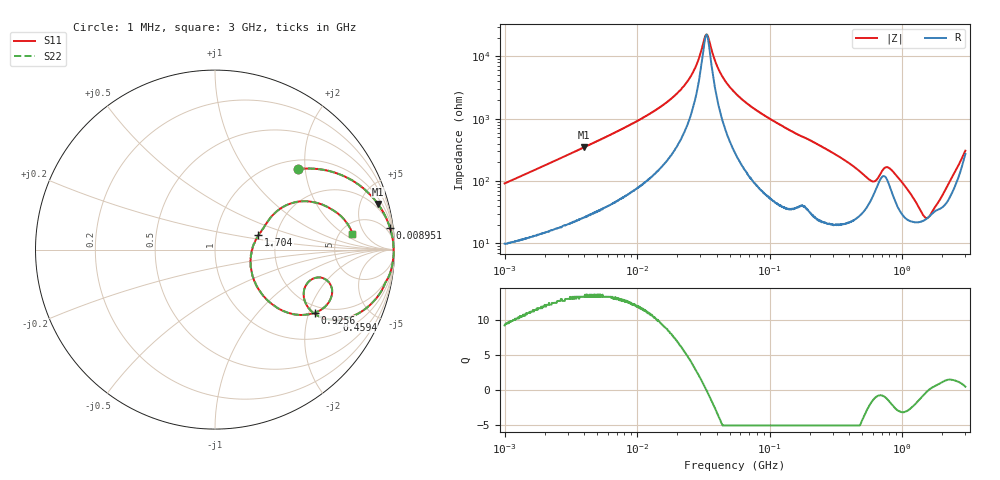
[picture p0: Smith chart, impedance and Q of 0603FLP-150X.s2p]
!s-Parameter Generated by FASTRON Sdn. Bhd.
!FASTRON P/N : 0603FLP-150X
!Keysight Technologies: E4991B_MY54100416_A.01.15
!Date: Tue Dec 02 13:15:56 2025
!Version  :Rev00  Tue Dec 02 13:15:56 2025
!Data & Calibration Information:
!Freq  S11  S21  S12  S22
!PortZ  Port1:50+j0  Port2:50+j0
!When reading reference impedance value at option line is always used.
! Remarks : This data is being provided solely for informational purposes.
# Hz S dB R 50
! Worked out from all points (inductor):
!   1601 points, 1 MHz to 3 GHz, reference 50 ohm
!   read as one part in series: L = 14.3 uH near 1.041 MHz
!   highest Q = 13.3 at 3.959 MHz (marker M1), where L = 13.9 uH
!   self-resonance near 33.37 MHz
!   S11 on the Smith chart (normalised r, x): 1 MHz: 1.20, +1.82; 8.951 MHz: 2, +16; 459.4 MHz: 1.52, -3.03; 925.6 MHz: 1.76, -2.18; 1.704 GHz: 1.61, +0.27; 3 GHz: 6.44, +2.85
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1000000  -3.85 44.2  -3.08 -39.6  -3.08 -39.6  -3.85 44.2
3804036  -0.55 16.3  -11.00 -69.4  -11.00 -69.4  -0.55 16.3
3959408  -0.52 15.7  -11.30 -70.0  -11.30 -70.0  -0.52 15.7
8950802  -0.15 7.0  -18.30 -78.4  -18.30 -78.4  -0.15 7.0
1.447069e7  -0.08 3.8  -23.40 -80.4  -23.40 -80.4  -0.08 3.8
2.435018e7  -0.05 1.3  -32.50 -76.5  -32.50 -76.5  -0.05 1.3
2.801249e7  -0.04 0.7  -37.30 -69.1  -37.30 -69.1  -0.04 0.7
3.337442e7  -0.04 0.0  -47.10 -0.1  -47.10 -0.1  -0.04 0.0
4.22235e7  -0.04 -1.0  -34.90 75.5  -34.90 75.5  -0.04 -1.0
5.504702e7  -0.04 -2.2  -28.30 81.7  -28.30 81.7  -0.04 -2.2
9.170654e7  -0.08 -5.1  -21.10 81.8  -21.10 81.8  -0.08 -5.1
2.083556e8  -0.35 -12.7  -13.10 73.5  -13.10 73.5  -0.35 -12.7
4.593788e8  -2.15 -30.0  -5.89 50.3  -5.89 50.3  -2.15 -30.0
6.018993e8  -5.09 -27.4  -4.93 26.9  -4.93 26.9  -5.09 -27.4
6.889699e8  -4.46 -15.0  -6.94 20.2  -6.94 20.2  -4.46 -15.0
7.925923e8  -3.13 -20.9  -7.37 35.5  -7.37 35.5  -3.13 -20.9
9.255909e8  -3.65 -32.4  -4.92 38.4  -4.92 38.4  -3.65 -32.4
1.153559e9  -6.69 -43.3  -2.67 25.6  -2.67 25.6  -6.69 -43.3
1.496395e9  -13.70 -17.2  -1.89 4.4  -1.89 4.4  -13.70 -17.2
1.704314e9  -11.90 18.3  -2.36 -6.0  -2.36 -6.0  -11.90 18.3
2.278218e9  -5.02 28.7  -4.80 -27.9  -4.80 -27.9  -5.02 28.7
3e9  -2.26 6.7  -12.00 -20.9  -12.00 -20.9  -2.26 6.7
